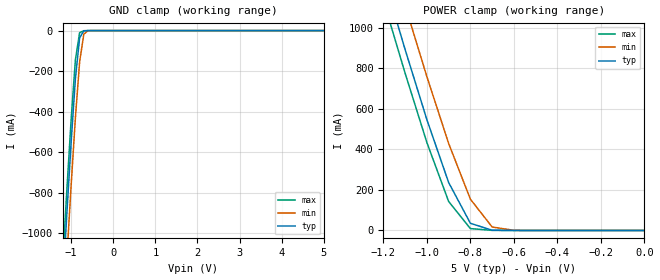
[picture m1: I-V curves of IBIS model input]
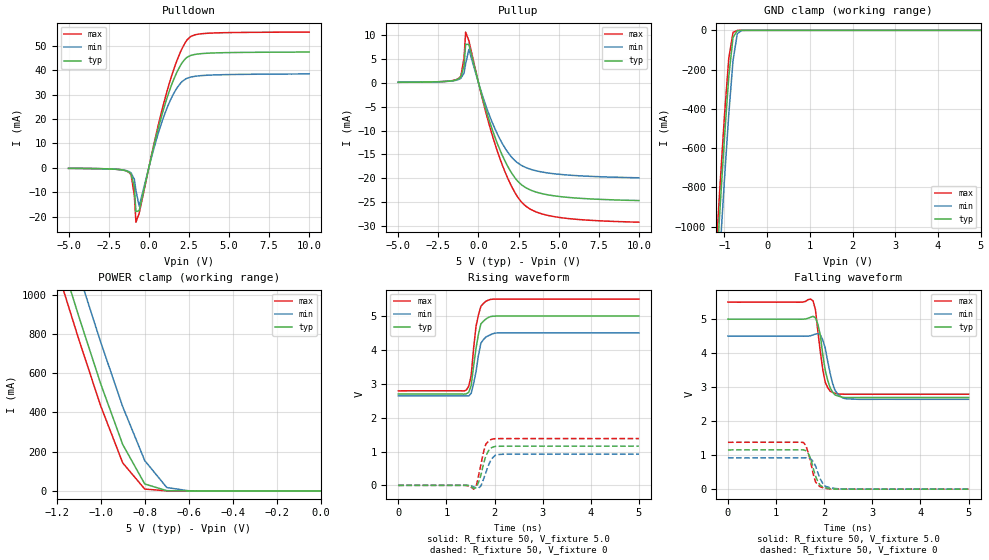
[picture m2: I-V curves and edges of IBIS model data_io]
| TSOP package & Commercial  operation.
[IBIS Ver]   3.2
[Comment Char]   |_char
[File name]   as7c1026b_tsopc.ibs
[File Rev]   1.0
[Date]   May 26, 2004 10:30:22 AM
[Source]
Alliance Semiconductor Corporation
[Notes]
This model  is for TSOP package & Commercial operation.
[Disclaimer]
Data is for modeling purpose only and is not guaranted.
This IBIS model is provided on an "AS IS" basis and Alliance Semiconductor makes
absolutely no warranty with respect to the information contained
herein.The entire risk as to quality and performance
is with the Customer. ACCORDINGLY, IN NO EVENT SHALL THE COMPANY BE
LIABLE FOR ANY DAMAGES, WHETHER IN CONTRACT OR TORT,INCLUDING ANY
LOST PROFITS OR OTHER INCIDENTAL, CONSEQUENTIAL, EXEMPLARY, OR
PUNITIVE DAMAGES ARISING OUT OF THE USE OR APPLICATION OF THE IBIS
model provided in this package.
[Copyright]
Alliance Semiconductor Corporation
| tsop Package & commercial operation
[Component]   AS7C1026B_TSOPC
Si_location Pin
Timing_location Pin
[Manufacturer]   Alliance Semiconductor Corporation
[Package]
R_pkg   321.15m   142.5m   499.8m
L_pkg   5.882nH   2.534nH   9.23nH
C_pkg   1.013pF   0.614pF   1.412pF
[Pin] signal_name   model_name
1   A4   input
2   A3   input
3   A2   input
4   A1   input
5   A0   input
6   NCE   input
7   IO0   data_io
8   IO1   data_io
9   IO2   data_io
10   IO3   data_io
11   VCC   POWER
12   GND   GND
13   IO4   data_io
14   IO5   data_io
15   IO6   data_io
16   IO7   data_io
17   NWE   input
18   A15   input
19   A14   input
20   A13   input
21   A12   input
22   NC   NC
23   NC   NC
24   A11   input
25   A10   input
26   A9   input
27   A8   input
28   NC   NC
29   IO8   data_io
30   IO9   data_io
31   IO10   data_io
32   IO11   data_io
33   VCC   POWER
34   GND   GND
35   IO12   data_io
36   IO13   data_io
37   IO14   data_io
38   IO15   data_io
39   NLB   input
40   NUB   input
41   NOE   input
42   A7   input
43   A6   input
44   A5   input
| Models and submodels in the file (2): input (Input), data_io (I/O)
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[Model]   input
Model_type Input
Vinh=2.2V
Vinl=0.8V
C_comp   4pF   4pF   4pF
[Model Spec]
[Temperature Range] 25   70   0
[Voltage Range]   5.0   4.5   5.5
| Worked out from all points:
|   GND clamp passes 1 mA (typ) near -0.67 V on its own axis
|   POWER clamp passes 1 mA (typ) near -0.68 V on its own axis
[GND Clamp]
-5V       -16.01A    -16.21A    -15.91A
-1.2V     -1.253A    -1.472A    -1.135A
-1.1V     -892.6mA   -1.11A     -775.9mA
-1V       -547.3mA   -759.1mA   -435mA
-900mV    -237.4mA   -430.4mA   -144.1mA
-800mV    -36.26mA   -154.9mA   -10.33mA
-700mV    -1.383mA   -17.31mA   -546.7uA
-600mV    -81.45uA   -732.3uA   -58.64uA
5V        292.5pA    38.81uA    -1.719nA
[POWER Clamp]
-5V       16.01A     16.21A     15.9A
-1.2V     1.252A     1.471A     1.135A
-1.1V     891.7mA    1.109A     775mA
-1V       546.1mA    758.3mA    433.5mA
-900mV    236.6mA    429.1mA    142.8mA
-800mV    35.4mA     154.3mA    9.383mA
-700mV    1.248mA    17.09mA    442.2uA
-600mV    85.03uA    719uA      72.84uA
0V        292.5pA    1.265nA    178.1pA
[Model]   data_io
Model_type I/O
Enable Active-High
Polarity Non-Inverting
Vinh=2.2V
Vinl=0.8V
Vref=1.728V
Vmeas=1.5V
Rref=168
Cref=30pF
C_comp   4pF   4pF   4pF
[Temperature Range] 25   70   0
[Voltage Range]   5.0   4.5   5.5
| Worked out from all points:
|   slope of the pulldown table from 0 to 0.75 V, typ, clamps not added: 37.5 ohm
|   slope of the pullup table from 0 to 0.75 V, typ, clamps not added: 86.3 ohm
|   GND clamp passes 1 mA (typ) near -0.67 V on its own axis
|   POWER clamp passes 1 mA (typ) near -0.68 V on its own axis
|   falling waveform, R_fixture 50, V_fixture 5.0: 20-80 % time 166ps typ, 174ps min, 152ps max; typ from 5 V to 2.7 V
|   falling waveform, R_fixture 50, V_fixture 0: 20-80 % time 154ps typ, 164ps min, 145ps max; typ from 1.16 V to 0.002 V
|   rising waveform, R_fixture 50, V_fixture 5.0: 20-80 % time 146ps typ, 141ps min, 134ps max; typ from 2.69 V to 5 V
|   rising waveform, R_fixture 50, V_fixture 0: 20-80 % time 139ps typ, 149ps min, 130ps max; typ from 0 V to 1.16 V
[Pullup]
-5V       80uA       70uA       70uA
-1.2V     863uA      707uA      969uA
-1.1V     1.172mA    910uA      1.369mA
-900mV    3.44mA     1.986mA    5.102mA
-800mV    8.002mA    3.941mA    10.56mA
-600mV    8.001mA    6.927mA    8.778mA
300mV     -3.74mA    -3.217mA   -4.145mA
1.1V      -12.04mA   -10.19mA   -13.54mA
2V        -18.52mA   -15.3mA    -21.23mA
2.7V      -21.38mA   -17.33mA   -25.01mA
4.7V      -23.63mA   -19.03mA   -27.98mA
10V       -24.63mA   -19.87mA   -29.15mA
[Pulldown]
-5V       -150uA     -150uA     -150uA
-1.2V     -1.84mA    -1.556mA   -1.973mA
-1.1V     -2.529mA   -2.05mA    -2.832mA
-900mV    -7.724mA   -4.62mA    -11.16mA
-800mV    -17.8mA    -9.214mA   -22.14mA
-600mV    -17.46mA   -15.57mA   -18.56mA
300mV     8.509mA    7.527mA    9.114mA
1.1V      27.83mA    23.89mA    30.48mA
1.8V      39.75mA    33.09mA    44.64mA
2.4V      45.28mA    36.68mA    52.42mA
3.6V      46.86mA    37.87mA    55mA
10V       47.36mA    38.41mA    55.51mA
[GND Clamp]
-5V       -16.01A    -16.21A    -15.91A
-1.2V     -1.253A    -1.472A    -1.135A
-1.1V     -892.6mA   -1.11A     -775.9mA
-1V       -547.3mA   -759.1mA   -435mA
-900mV    -237.4mA   -430.4mA   -144.1mA
-800mV    -36.26mA   -154.9mA   -10.33mA
-700mV    -1.383mA   -17.31mA   -546.7uA
-600mV    -81.45uA   -732.3uA   -58.64uA
5V        292.5pA    38.81uA    -1.719nA
[POWER Clamp]
-5V       16.01A     16.21A     15.9A
-1.2V     1.252A     1.471A     1.135A
-1.1V     891.7mA    1.109A     775mA
-1V       546.1mA    758.3mA    433.5mA
-900mV    236.6mA    429.1mA    142.8mA
-800mV    35.4mA     154.3mA    9.383mA
-700mV    1.248mA    17.09mA    442.2uA
-600mV    85.03uA    719uA      72.84uA
0V        292.5pA    1.265nA    178.1pA
[Falling Waveform]
R_fixture=50
V_fixture=5.0
V_fixture_min=4.5
V_fixture_max=5.5
0s        5V         4.5V       5.5V
1.768ns   5.082V     4.535V     5.534V
1.818ns   5.035V     4.558V     5.27V
1.869ns   4.848V     4.577V     4.632V
1.97ns    3.957V     4.391V     3.521V
2.02ns    3.502V     4.152V     3.147V
2.172ns   2.857V     3.121V     2.848V
2.273ns   2.747V     2.816V     2.805V
2.424ns   2.694V     2.665V     2.792V
5ns       2.696V     2.643V     2.791V
[Falling Waveform]
R_fixture=50
V_fixture=0
V_fixture_min=0
V_fixture_max=0
0s        1.155V     920.1mV    1.378V
1.566ns   1.159V     924.2mV    1.373V
1.616ns   1.134V     924.9mV    1.297V
1.717ns   908.6mV    896.5mV    814.1mV
1.768ns   630.4mV    818.4mV    466.7mV
1.818ns   391.8mV    691.6mV    214.3mV
1.919ns   106.7mV    297.7mV    69.14mV
2.02ns    45.89mV    88.54mV    25.45mV
2.424ns   2.522mV    4.679mV    2.356mV
5ns       2.452mV    2.344mV    2.584mV
[Rising Waveform]
R_fixture=50
V_fixture=5.0
V_fixture_min=4.5
V_fixture_max=5.5
0s        2.694V     2.642V     2.789V
1.414ns   2.701V     2.64V      2.813V
1.465ns   2.746V     2.636V     2.925V
1.515ns   2.949V     2.719V     3.244V
1.616ns   4.042V     3.356V     4.696V
1.667ns   4.461V     3.841V     5.033V
1.717ns   4.764V     4.195V     5.283V
1.869ns   4.95V      4.412V     5.463V
2.071ns   4.996V     4.497V     5.496V
5ns       4.996V     4.497V     5.496V
[Rising Waveform]
R_fixture=50
V_fixture=0
V_fixture_min=0
V_fixture_max=0
0s        0V         0V         0V
1.364ns   3.513mV    2.98mV     3.753mV
1.566ns   -84.79mV   -43.58mV   -110.8mV
1.616ns   -70.03mV   -68.86mV   -45.51mV
1.717ns   298.9mV    -19.06mV   612.7mV
1.818ns   866.3mV    366.9mV    1.215V
1.919ns   1.103V     736.2mV    1.35V
1.97ns    1.132V     830.8mV    1.369V
2.273ns   1.157V     923mV      1.381V
5ns       1.157V     922.5mV    1.381V
[Ramp]
R_load=50
dV/dt_r   6.942E-1/1.333E-10   5.535E-1/1.489E-10   8.285E-1/1.220E-10
dV/dt_f   1.383E+0/1.624E-10   1.114E+0/1.663E-10   1.625E+0/1.452E-10
|[End   data_io
